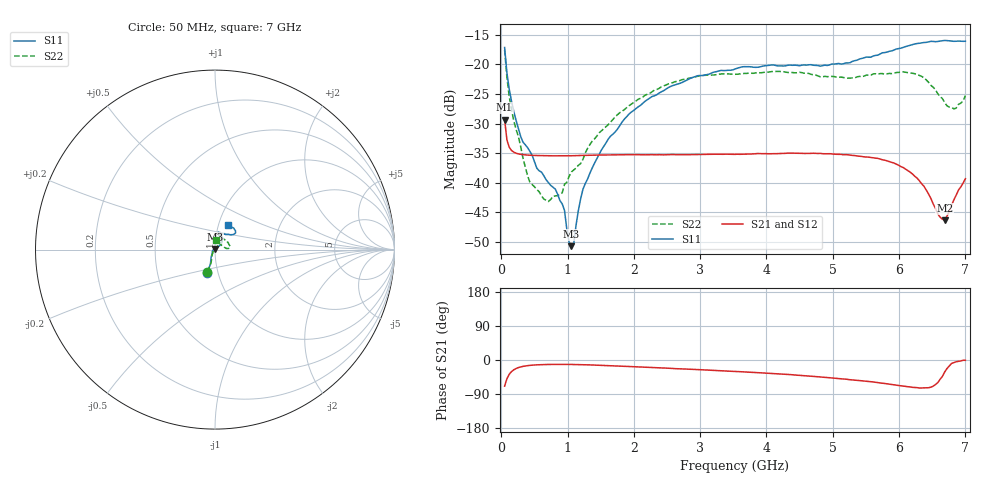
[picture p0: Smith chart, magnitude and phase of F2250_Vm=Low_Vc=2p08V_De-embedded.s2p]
! Integrated Device Technology
! Corporate Headquarters
! 6024 Silver Creek Valley Road
! San Jose, CA 95138  USA
! Phone:  1-408-284-8200
! Toll Free:  1-800-223-1366
! Webpage:  http://www.idt.com/
! Timing and RF Division
! 515 Groton Road, Suite 102
! Westford, MA 01886-6024
! Device:  F2250
! Description: Voltage Variable RF Attenuator
! Frequency:  50.0 -  6000.00 MHz
! Package:  3x3 mm Thin QFN Plastic Package: 16 pin
! Ports:  2 RF, 3 DC
!  Pin  1  = GND
!  Pin  2  = NC
!  Pin  3  = RF1  = Port 1
!  Pin  4  = NC
!  Pin  5  = GND
!  Pin  6  = GND
!  Pin  7  = GND
!  Pin  8  = GND
!  Pin  9  = NC
!  Pin 10  = RF2  = Port 2
!  Pin 11  = NC
!  Pin 12  = GND
!  Pin 13  = GND
!  Pin 14  = VCNTRL
!  Pin 15  = VDD
!  Pin 16  = VMODE
! Vcntrl:  2.080 Volts
! Vmode:  +0.000 Volts
! Vdd:  +3.30  Volts
! Current:  1.180 mA
! Data:  The device was measured on a the F2250 evaluation board which has
!  individual transmission lines to the RF pins.  Data was collected
!  using a calibrated network analyzer.  The evaluation board was
!  de-embedded using a TRL calibration technique.
!  The reference plane is the edge of the package pin.
! Misc:  SN 10
!  Action Tracker AT0258
! Date Measured:  2014-11-26
! Date:  2015-10-15  MJV
! Note:
!  Integrated Device Technology supplies this data as a sample of measured
!  data at the package pin for this product.  Your particular data for this
!  product may vary.
!  Data was taken at 25 degrees C.
!  Integrated Device Technology reserves the right to change this data at anytime.
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# GHz S dB R 50
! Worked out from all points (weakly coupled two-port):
!   201 points, 50 MHz to 7 GHz, reference 50 ohm
!   highest |S21| = -29.33 dB at 50 MHz (marker M1); lowest = -46.3 dB at 6.687 GHz (marker M2)
!   lowest |S11| = -50.7 dB at 1.058 GHz (marker M3), VSWR 1.01, Z = 49.8 + j0.244 ohm
!   |S11| at or under -10 dB: start of sweep to end of sweep
!   |S22| runs from -43.1 to -17.6 dB; largest |S21 - S12| = 6.1e-05
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0.05  -17.18 -108.6  -29.33 -68.9  -29.33 -68.9  -17.59 -109.5
0.08475  -21.44 -107.4  -32.76 -49.5  -32.76 -49.5  -22.21 -106.4
0.189  -28.01 -119.7  -34.83 -25.8  -34.84 -25.8  -29.57 -118.1
0.29325  -32.21 -127.7  -35.20 -18.2  -35.20 -18.2  -33.93 -124.1
0.43225  -34.71 -144.6  -35.35 -14.1  -35.35 -14.1  -39.92 -157.2
0.71025  -39.95 -168.6  -35.43 -11.8  -35.44 -11.8  -43.14 142.9
0.91875  -43.55 158.1  -35.45 -11.6  -35.45 -11.6  -41.68 106.8
0.9535  -44.64 170.3  -35.45 -11.6  -35.44 -11.6  -40.25 107.5
1.023  -49.99 143.9  -35.44 -11.7  -35.44 -11.7  -38.90 88.9
1.05775  -50.68 123.3  -35.43 -11.8  -35.43 -11.8  -38.16 84.3
1.0925  -50.31 89.0  -35.42 -11.9  -35.42 -11.9  -37.84 79.3
1.162  -44.69 56.7  -35.40 -12.1  -35.41 -12.1  -37.04 68.8
1.2315  -41.08 44.3  -35.37 -12.3  -35.37 -12.3  -36.04 60.8
1.6485  -32.12 42.0  -35.29 -14.9  -35.29 -14.9  -29.76 52.4
2.37825  -24.87 47.3  -35.26 -20.7  -35.26 -20.7  -24.08 50.7
3.525  -20.80 72.5  -35.20 -30.1  -35.19 -30.1  -21.69 71.6
4.7065  -20.17 72.4  -35.01 -43.2  -35.01 -43.2  -21.78 70.5
5.85325  -17.82 40.4  -36.42 -63.7  -36.42 -63.8  -21.55 19.7
6.33975  -16.40 41.0  -40.15 -73.8  -40.16 -73.8  -22.04 5.6
6.68725  -15.99 48.8  -46.32 -31.8  -46.32 -31.5  -26.45 25.7
6.861  -16.12 55.1  -42.07 -4.6  -42.03 -4.6  -27.40 58.4
7  -16.12 63.3  -39.30 -0.8  -39.27 -0.9  -25.29 85.5
